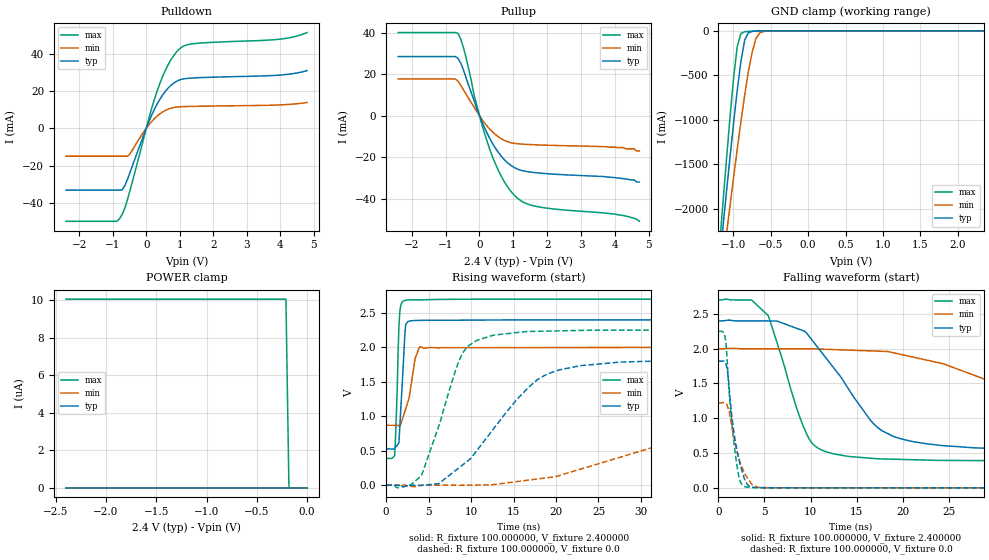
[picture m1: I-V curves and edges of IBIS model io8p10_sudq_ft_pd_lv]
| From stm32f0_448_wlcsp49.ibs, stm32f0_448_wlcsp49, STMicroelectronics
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|   Model io8p10_sudq_ft_pd_lv
[Model]  io8p10_sudq_ft_pd_lv
Model_type I/O
Polarity   Non-Inverting
Enable   Active-Low
Vinl =   0.720000V
Vinh =   1.680000V
Vmeas =  1.200000V
Cref =   50.000000pF
Rref =   100.000000M
Vref =   0.0V
C_comp   1.970100pF   1.887900pF   2.069400pF
[Temperature Range]   25.000000   0.125000k   -40.000000
[Pullup Reference]   2.400000V   2.000000V   2.700000V
[Pulldown Reference]   0.0V   0.0V   0.0V
[POWER Clamp Reference]   2.400000V   2.000000V   2.700000V
[GND Clamp Reference]   0.0V   0.0V   0.0V
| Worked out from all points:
|   slope of the pulldown table from 0 to 0.36 V, typ, clamps not added: 25.5 ohm
|   slope of the pullup table from 0 to 0.36 V, typ, clamps not added: 28.4 ohm
|   GND clamp passes 1 mA (typ) near -0.64 V on its own axis
|   rising waveform, R_fixture 100.000000, V_fixture 2.400000: 20-80 % time 501ps typ, 1.06ns min, 337ps max; typ from 0.525 V to 2.4 V
|   rising waveform, R_fixture 100.000000, V_fixture 0.0: 20-80 % time 7.37ns typ, 21.8ns min, 3.53ns max; typ from 0 V to 1.82 V
|   falling waveform, R_fixture 100.000000, V_fixture 2.400000: 20-80 % time 6.27ns typ, 17.5ns min, 3.34ns max; typ from 2.4 V to 0.525 V
|   falling waveform, R_fixture 100.000000, V_fixture 0.0: 20-80 % time 1.15ns typ, 1.39ns min, 910ps max; typ from 1.82 V to 0 V
[Pulldown]
|Voltage   I(typ)   I(min)   I(max)
-2.4V     -33.16mA   -14.98mA   -49.86mA
-880mV    -33.16mA   -14.98mA   -49.86mA
-800mV    -33.16mA   -14.98mA   -48.55mA
-640mV    -30.75mA   -14.98mA   -42.76mA
-480mV    -23.43mA   -13.57mA   -32.92mA
80mV      3.651mA    1.905mA    5.506mA
400mV     15.37mA    7.665mA    23.73mA
720mV     22.75mA    10.69mA    36.23mA
1.04V     26.18mA    11.57mA    43.27mA
1.52V     27.09mA    11.81mA    45.55mA
4V        28.55mA    12.55mA    47.81mA
4.8V      30.9mA     13.81mA    51.31mA
[Pullup]
|Voltage   I(typ)   I(min)   I(max)
-2.4V     28.56mA    17.75mA    40.16mA
-720mV    28.56mA    17.75mA    40.16mA
-640mV    27.85mA    16.83mA    39.87mA
-480mV    22.39mA    12.66mA    33.22mA
-80mV     3.427mA    2.067mA    4.957mA
160mV     -6.219mA   -3.715mA   -9.137mA
320mV     -11.51mA   -6.781mA   -16.98mA
720mV     -21mA      -11.8mA    -31.53mA
1.12V     -25.77mA   -13.54mA   -39.82mA
1.76V     -27.69mA   -14.12mA   -44.07mA
4V        -29.9mA    -15.2mA    -47.5mA
4.72V     -32mA      -17mA      -51mA
[GND_clamp]
|Voltage   I(typ)   I(min)   I(max)
-2.4V     -9.788A    -9.782A    -9.734A
-1.2V     -2.718A    -3.021A    -2.568A
-1.15V    -2.29A     -2.675A    -2.036A
-1.1V     -1.868A    -2.333A    -1.515A
-1.05V    -1.454A    -1.995A    -1.012A
-950mV    -674.5mA   -1.337A    -180.6mA
-900mV    -345.2mA   -1.023A    -29.74mA
-850mV    -106.4mA   -726mA     -10.14mA
-750mV    -6.411mA   -244mA     -4.042mA
-700mV    -2.572mA   -88.62mA   -2.346mA
-600mV    -429.6uA   -7.75mA    -383.5uA
2.35V     59.77uA    46.33uA    66.89uA
[POWER_clamp]
|Voltage   I(typ)   I(min)   I(max)
-2.4V     0A         0A         10.06uA
-210mV    0A         0A         10.06uA
-180mV    0A         0A         0A
0V        0A         0A         0A
[Ramp]
| variable   typ   min   max
dV/dt_r  1.09206/7.36205n   0.73212/21.76780n   1.34880/3.52140n
dV/dt_f  1.12434/6.26286n   0.67629/17.46251n   1.38699/3.33301n
R_load = 100.000000
[Rising Waveform]
R_fixture= 100.000000
V_fixture= 2.400000
V_fixture_min= 2.000000
V_fixture_max= 2.700000
|time   V(typ)   V(min)   V(max)
0s        524.8mV    868.7mV    387.2mV
1.001ns   532.8mV    867mV      426.6mV
1.301ns   578.6mV    865.5mV    1.387V
1.502ns   616.5mV    864.9mV    2.303V
1.702ns   1.053V     875.4mV    2.602V
2.102ns   1.953V     1.031V     2.676V
2.302ns   2.331V     1.108V     2.683V
3.403ns   2.389V     1.835V     2.689V
4.004ns   2.392V     2.014V     2.689V
49.85ns   2.399V     1.999V     2.699V
[Rising Waveform]
R_fixture= 100.000000
V_fixture= 0.0
V_fixture_min= 0.0
V_fixture_max= 0.0
|time   V(typ)   V(min)   V(max)
0s        1.768nV    15.89nV    1.355nV
2.803ns   -3.26mV    -14.06mV   -1.551mV
4.204ns   -1.822mV   -2.484mV   153.2mV
6.206ns   24.43mV    -1.172mV   860.8mV
8.809ns   274.4mV    -1.373mV   1.867V
12.61ns   812.3mV    7.914mV    2.175V
17.82ns   1.532V     89.58mV    2.232V
23.02ns   1.735V     237.2mV    2.246V
50.05ns   1.82V      1.08V      2.248V
99.7ns    1.82V      1.221V     2.248V
[Falling Waveform]
R_fixture= 100.000000
V_fixture= 2.400000
V_fixture_min= 2.000000
V_fixture_max= 2.700000
|time   V(typ)   V(min)   V(max)
0s        2.399V     1.999V     2.699V
3.604ns   2.399V     1.998V     2.698V
5.405ns   2.398V     1.998V     2.475V
9.61ns    2.218V     1.997V     767.5mV
12.61ns   1.708V     1.986V     485.9mV
17.62ns   835.2mV    1.963V     416.1mV
24.42ns   606.3mV    1.782V     394.4mV
31.83ns   557.1mV    1.421V     389.7mV
47.25ns   529mV      987.2mV    387.3mV
99.7ns    524.8mV    868.7mV    387.2mV
[Falling Waveform]
R_fixture= 100.000000
V_fixture= 0.0
V_fixture_min= 0.0
V_fixture_max= 0.0
|time   V(typ)   V(min)   V(max)
0s        1.82V      1.221V     2.248V
700.7ps   1.8V       1.221V     2.179V
800.8ps   1.783V     1.214V     2.096V
1.001ns   1.653V     1.163V     1.703V
1.401ns   1.09V      921.9mV    991.5mV
1.802ns   688.2mV    647.3mV    514.6mV
2.302ns   364.8mV    386.2mV    116.7mV
2.903ns   104.8mV    188.7mV    16.24mV
4.705ns   2.13mV     3.846mV    2.055mV
49.85ns   1.768nV    15.89nV    1.355nV
